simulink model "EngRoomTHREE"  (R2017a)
settings: Solver=VariableStepAuto  StartTime=0.0  StopTime=10.0  RelTol=1e-3
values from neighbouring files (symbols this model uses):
  EngDat = engine_pre()    [run_master.m]    (also in engine_pre.m = [MCR1, BSFC1, x)
undefined symbols (not defined in the file or in its folder): num

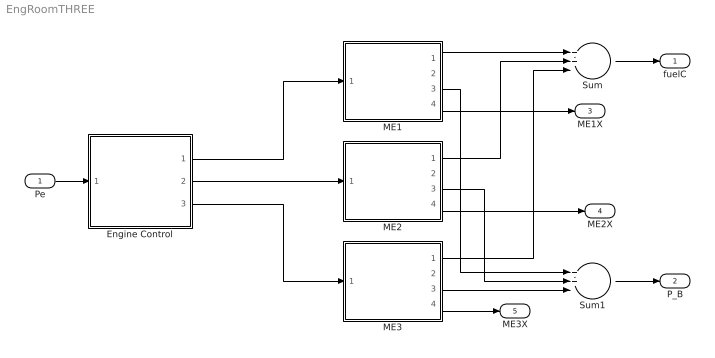
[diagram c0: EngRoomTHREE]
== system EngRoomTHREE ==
  Pe : Inport
  Engine Control : MATLAB Function  TreatAsAtomicUnit=on
  ME1 : MATLAB Function  TreatAsAtomicUnit=on
  ME2 : MATLAB Function  TreatAsAtomicUnit=on
  ME3 : MATLAB Function  TreatAsAtomicUnit=on
  Sum : Sum  Inputs=3
  Sum1 : Sum  Inputs=3
  fuelC : Outport
  P_B : Outport  Port=2
  ME1X : Outport  Port=3
  ME2X : Outport  Port=4
  ME3X : Outport  Port=5
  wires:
  Pe/1 -> Engine Control/1(Pe)
  Engine Control/1(P1) -> ME1/1("Pb ")
  Engine Control/2(P2) -> ME2/1("Pb ")
  Engine Control/3(P3) -> ME3/1("Pb ")
  Sum/1 -> fuelC/1
  ME1/1(fuel_cons) -> Sum/1
  ME2/1(fuel_cons) -> Sum/2
  ME3/1(fuel_cons) -> Sum/3
  ME3/3(Pb) -> Sum1/3
  ME2/3(Pb) -> Sum1/2
  ME1/3(Pb) -> Sum1/1
  Sum1/1 -> P_B/1
  ME1/4(x) -> ME1X/1
  ME2/4(x) -> ME2X/1
  ME3/4(x) -> ME3X/1

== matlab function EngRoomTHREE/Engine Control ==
function [P1, P2, P3] = fcn(Pe,EngDat)
%take in the total propulsive powering need and Machinery data

%find the optimal settings so that each engine runs close to optimum
%output the load (and rpm) for each engine

%Pe is the required effective power to overcome resistance, the break power
%needed from the engineroom depends on the efficiency of the propulsion
%system, which in turn depends on the configuration of the engines and
%propulsors

% EngDat=([MCR,BSFC,x])

%Read data about the engines from the workspace

%capacity of each engine
PMCR1=EngDat(1,1);
PMCR2=EngDat(2,1);
PMCR3=EngDat(3,1);

%pre-set to 0
P1=0;
P2=0;
P3=0;
%% Convert Pe into Pb required from the machinery
eta_D = 0.55;
eta_M = 0.95*0.98;
eta_T = eta_D* eta_M;   %Total efficiency
Pb = (Pe/eta_T); %kW

  if Pb<=PMCR3 % If the required load is less than capacity of eng 3
            P1=0; 
            P2=0;
            P3=Pb;
            return
  elseif Pb<=PMCR2 % If the required load is less than capacity of eng 2
            P1=0;
            P2=Pb;
            P3=0;
            return
  elseif Pb<=PMCR1
            P1=Pb;
            P2=0;
            P3=0;   
            return
  elseif Pb<=(PMCR3+PMCR2)
            load=Pb/(PMCR2+PMCR3);
            P2=load*PMCR2;
            P3=load*PMCR3;
            return
  elseif Pb<=(PMCR1+PMCR3)
            load=Pb/(PMCR1+PMCR3);
            P1=load*PMCR1;
            P3=load*PMCR3;
            return
  elseif Pb<=(PMCR1+PMCR2)
            load=Pb/(PMCR1+PMCR2);
            P1=load*PMCR1;
            P2=load*PMCR2;
            return
  else 
            load=Pb/(PMCR1+PMCR2+PMCR3);
            P1=load*PMCR1;
            P2=load*PMCR2;
            P3=load*PMCR3;          
  end
  
 
end

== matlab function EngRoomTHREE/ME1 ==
function [fuel_cons,nshaft, Pb, x] = fcn(Pb, num, EngDat)


PMCR=EngDat(1,1);
x = Pb/PMCR; %percentage of maximum
BSFC=EngDat(1,2); %g/kWh
delta_BSFC = 6610.6*x^6 - 20524*x^5 + 23791*x^4 - 11985*x^3 + 1803.2*x^2 + 340.12*x - 36.733;


fuel_cons = (delta_BSFC+BSFC)*Pb/1000; %kg/h

nshaft=neng;


end

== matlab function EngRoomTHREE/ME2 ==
function [fuel_cons,nshaft, Pb, x] = fcn(Pb, num, EngDat)

PMCR=EngDat(2,1);
x = Pb/PMCR; %percentage of maximum
BSFC=EngDat(2,2); %g/kWh
delta_BSFC = 6610.6*x^6 - 20524*x^5 + 23791*x^4 - 11985*x^3 + 1803.2*x^2 + 340.12*x - 36.733;


fuel_cons = (delta_BSFC+BSFC)*Pb/1000; %kg/h

nshaft=neng;


end

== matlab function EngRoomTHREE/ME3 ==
function [fuel_cons,nshaft, Pb, x] = fcn(Pb, num, EngDat)


PMCR=EngDat(3,1);
x = Pb/PMCR; %percentage of maximum
BSFC=EngDat(3,2); %g/kWh
delta_BSFC = 6610.6*x^6 - 20524*x^5 + 23791*x^4 - 11985*x^3 + 1803.2*x^2 + 340.12*x - 36.733;


fuel_cons = (delta_BSFC+BSFC)*Pb/1000; %kg/h

nshaft=neng;


end
